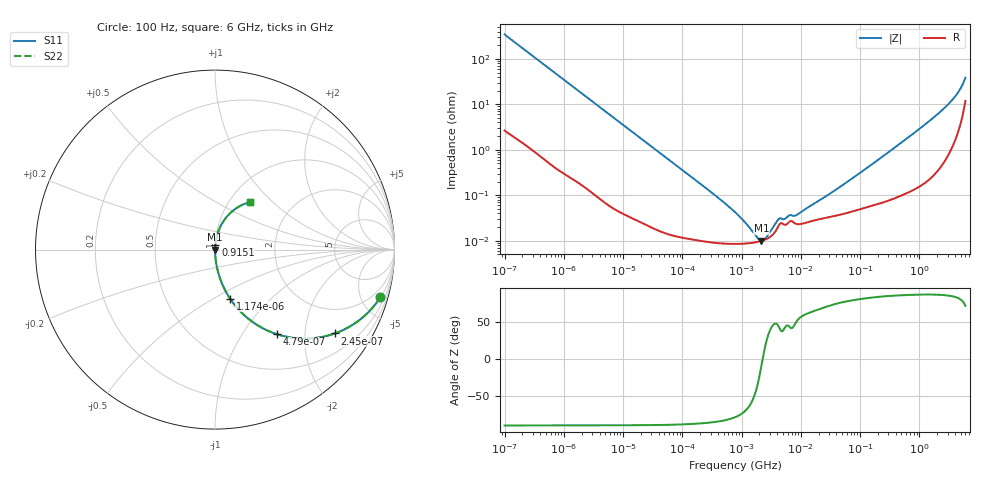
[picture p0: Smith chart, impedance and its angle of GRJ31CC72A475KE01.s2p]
!Murata Part Number: GRJ31CC72A475KE01
!These Parameters are Measured in Series Mode Connection
!Data Generated on Jun 19, 2026
!  o--ll--o
!Port1  Port2
!  o------o
!Operation Temp=25[degC], DC Bias Voltage=0[V]
!Freq. Start=100[Hz] Stop=6[GHz] 401[Steps]
# Hz S RI R 50
!Freq.(Hz) S11(Real) S11(Imag) S21(Real) S21(Imag) S12(Real) S12(Imag) S22(Real) S22(Imag)
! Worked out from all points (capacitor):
!   401 points, 100 Hz to 6 GHz, reference 50 ohm
!   read as one part in series: C = 4.59 uF near 109 Hz
!   lowest |Z| = 9.98 mohm at 2.169 MHz (marker M1)
!   series resonance near 2.269 MHz, so ESL is about 1.1 nH
!   S11 on the Smith chart (normalised r, x): 100 Hz: 1.05, -6.93; 245 Hz: 1.02, -2.84; 479 Hz: 1.01, -1.46; 1.174 kHz: 1.01, -0.60; 915.1 MHz: 1.00, +0.05; 6 GHz: 1.24, +0.74
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100  0.9213 -0.2655  0.0787 0.2655  0.0787 0.2655  0.9213 -0.2655
150  0.8412 -0.3616  0.1588 0.3616  0.1588 0.3616  0.8412 -0.3616
245  0.6674 -0.467  0.3326 0.467  0.3326 0.467  0.6674 -0.467
479  0.3478 -0.4722  0.6522 0.4722  0.6522 0.4722  0.3478 -0.4722
750  0.1807 -0.3807  0.8193 0.3807  0.8193 0.3807  0.1807 -0.3807
1174  0.0839 -0.2729  0.9161 0.2729  0.9161 0.2729  0.0839 -0.2729
2008  0.0313 -0.1694  0.9687 0.1694  0.9687 0.1694  0.0313 -0.1694
6433  0.00355 -0.0548  0.9964 0.0548  0.9964 0.0548  0.00355 -0.0548
40335  0.000243 -0.00887  0.9998 0.00887  0.9998 0.00887  0.000243 -0.00887
774597  8.48e-05 -0.000416  0.9999 0.000416  0.9999 0.000416  8.48e-05 -0.000416
1813585  9.31e-05 -7.34e-05  0.9999 7.34e-05  0.9999 7.34e-05  9.31e-05 -7.34e-05
2169299  9.87e-05 -1.47e-05  0.9999 1.47e-05  0.9999 1.47e-05  9.87e-05 -1.47e-05
2594782  0.000108 4.44e-05  0.9999 -4.44e-05  0.9999 -4.44e-05  0.000108 4.44e-05
4246196  0.000217 0.000208  0.9998 -0.000208  0.9998 -0.000208  0.000217 0.000208
8311524  0.000234 0.000275  0.9998 -0.000275  0.9998 -0.000275  0.000234 0.000275
1.555665e7  0.000271 0.000553  0.9997 -0.000553  0.9997 -0.000553  0.000271 0.000553
4.983056e7  0.000384 0.0016  0.9996 -0.0016  0.9996 -0.0016  0.000384 0.0016
3.124326e8  0.000854 0.00911  0.9991 -0.00911  0.9991 -0.00911  0.000854 0.00911
9.150511e8  0.00212 0.0262  0.9979 -0.0262  0.9979 -0.0262  0.00212 0.0262
3.065283e9  0.0171 0.0971  0.9829 -0.0971  0.9829 -0.0971  0.0171 0.0971
4.586474e9  0.0567 0.1718  0.9433 -0.1718  0.9433 -0.1718  0.0567 0.1718
6e9  0.1944 0.2653  0.8056 -0.2653  0.8056 -0.2653  0.1944 0.2653
